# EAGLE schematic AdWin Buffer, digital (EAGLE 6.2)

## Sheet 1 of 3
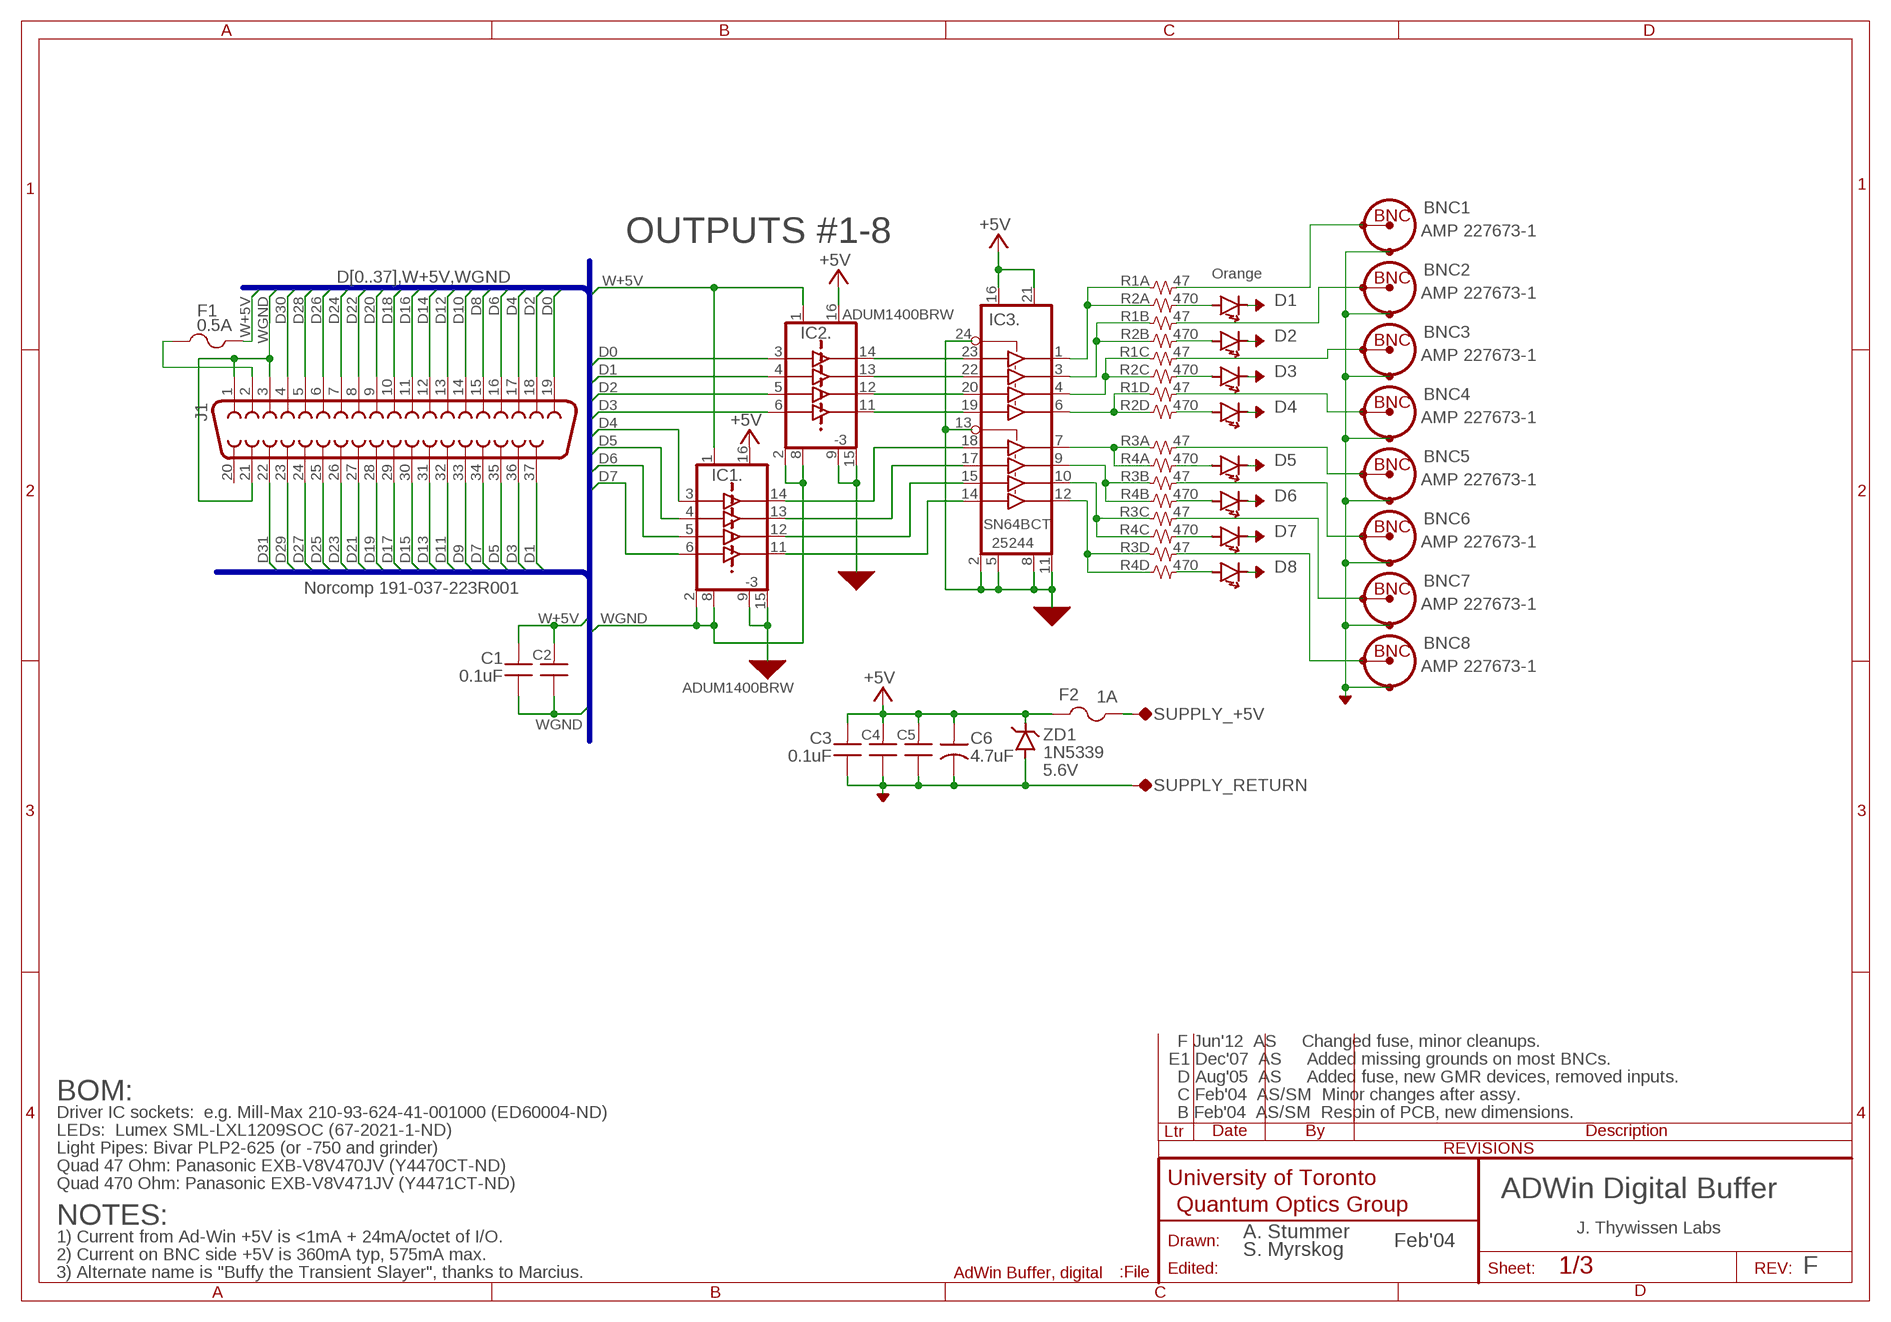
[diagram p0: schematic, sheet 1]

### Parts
BNC1  AMP 227673-1  CONN-BNC-TYPE1VERT  [CONN-BNC-AMP-TYPE1VERT]
BNC2  AMP 227673-1  CONN-BNC-TYPE1VERT  [CONN-BNC-AMP-TYPE1VERT]
BNC3  AMP 227673-1  CONN-BNC-TYPE1VERT  [CONN-BNC-AMP-TYPE1VERT]
BNC4  AMP 227673-1  CONN-BNC-TYPE1VERT  [CONN-BNC-AMP-TYPE1VERT]
BNC5  AMP 227673-1  CONN-BNC-TYPE1VERT  [CONN-BNC-AMP-TYPE1VERT]
BNC6  AMP 227673-1  CONN-BNC-TYPE1VERT  [CONN-BNC-AMP-TYPE1VERT]
BNC7  AMP 227673-1  CONN-BNC-TYPE1VERT  [CONN-BNC-AMP-TYPE1VERT]
BNC8  AMP 227673-1  CONN-BNC-TYPE1VERT  [CONN-BNC-AMP-TYPE1VERT]
C1  0.1uF  CAP-V-0805  [0805]
C2  0.1uF  CAP-V-0805  [0805]
C3  0.1uF  CAP-V-0805  [0805]
C4  0.1uF  CAP-V-0805  [0805]
C5  0.1uF  CAP-V-0805  [0805]
C6  4.7uF  CAP-POL-EIA-B  [EIA-B]
D1  LED-1209  [1209]
D2  LED-1209  [1209]
D3  LED-1209  [1209]
D4  LED-1209  [1209]
D5  LED-1209  [1209]
D6  LED-1209  [1209]
D7  LED-1209  [1209]
D8  LED-1209  [1209]
F1  0.5A  FUSE-5X20-4  [FUSE]
F2  1A  FUSE-5X20-4  [FUSE]
IC1  ADUM1400BRW  ISOLATOR,QUADTTLSOIC-16W  [SOIC-16W]
IC2  ADUM1400BRW  ISOLATOR,QUADTTLSOIC-16W  [SOIC-16W]
IC3  SN64BCT25244NT  LOGIC,BUFFER:64BCT2544(OCTAL)NT  [DIL24]
J1  Norcomp 191-037-223R001  CONN:DB37V  [CONN:DB37-VERT]
R1  47  R-4PAK-0603  [PANASONIC_EXB-V8V(QUAD-R-PACK)]
R2  470  R-4PAK-0603  [PANASONIC_EXB-V8V(QUAD-R-PACK)]
R3  47  R-4PAK-0603  [PANASONIC_EXB-V8V(QUAD-R-PACK)]
R4  470  R-4PAK-0603  [PANASONIC_EXB-V8V(QUAD-R-PACK)]
SUPPLY_+5V  TP-HOLE-0.042  [TP-HOLE]
SUPPLY_RETURN  TP-HOLE-0.042  [TP-HOLE]
ZD1  1N5339  ZENER-EIA-B  [EIA-B]

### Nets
+5V [PowerA]: C3.2 C4.2 C5.2 C6.2(POS) F2.1A IC1.16(.:VDDOUT) IC2.16(.:VDDOUT) IC3.16(.:VDD1) IC3.21(.:VDD2) ZD1.2(C) ; also sheet 2,3
AGND [PowerA]: BNC1.SHIELD BNC2.SHIELD BNC3.SHIELD BNC4.SHIELD BNC5.SHIELD BNC6.SHIELD BNC7.SHIELD BNC8.SHIELD C3.1 C4.1 C5.1 C6.1(NEG) D1.K(C) D2.K(C) D3.K(C) D4.K(C) D5.K(C) D6.K(C) D7.K(C) D8.K(C) IC1.9(.:COM1OUT) IC1.15(.:COM2OUT) IC2.9(.:COM1OUT) IC2.15(.:COM2OUT) IC3.2(.:COM1) IC3.5(.:COM2) IC3.8(.:COM3) IC3.11(.:COM4) IC3.13(.:EN-58) IC3.24(.:EN-14) SUPPLY_RETURN.P$1(TP) ZD1.1(A) ; also sheet 2,3
D0: IC2.3(IN) J1.19
D1: IC2.4(IN) J1.37
D2: IC2.5(IN) J1.18
D3: IC2.6(IN) J1.36
D4: IC1.3(IN) J1.17
D5: IC1.4(IN) J1.35
D6: IC1.5(IN) J1.16
D7: IC1.6(IN) J1.34
D8: J1.15 ; also sheet 2
D9: J1.33 ; also sheet 2
D10: J1.14 ; also sheet 2
D11: J1.32 ; also sheet 2
D12: J1.13 ; also sheet 2
D13: J1.31 ; also sheet 2
D14: J1.12 ; also sheet 2
D15: J1.30 ; also sheet 2
D16: J1.11 ; also sheet 3
D17: J1.29 ; also sheet 3
D18: J1.10 ; also sheet 3
D19: J1.28 ; also sheet 3
D20: J1.9 ; also sheet 3
D21: J1.27 ; also sheet 3
D22: J1.8 ; also sheet 3
D23: J1.26 ; also sheet 3
D24: J1.7 ; also sheet 3
D25: J1.25 ; also sheet 3
D26: J1.6 ; also sheet 3
D27: J1.24 ; also sheet 3
D28: J1.5 ; also sheet 3
D29: J1.23 ; also sheet 3
D30: J1.4 ; also sheet 3
D31: J1.22 ; also sheet 3
N$1: IC2.14(Q) IC3.23(1:IN)
N$2: IC2.13(Q) IC3.22(2:IN)
N$3: IC2.12(Q) IC3.20(3:IN)
N$4: IC2.11(Q) IC3.19(4:IN)
N$7: IC1.11(Q) IC3.14(8:IN)
N$10: IC3.6(4:Q) R1.4A R2.4A
N$11: IC3.4(3:Q) R1.3A R2.3A
N$12: IC3.3(2:Q) R1.2A R2.2A
N$13: IC3.1(1:Q) R1.1A R2.1A
N$14: IC3.7(5:Q) R3.1A R4.1A
N$15: IC3.9(6:Q) R3.2A R4.2A
N$16: IC1.12(Q) IC3.15(7:IN)
N$17: IC1.13(Q) IC3.17(6:IN)
N$18: IC1.14(Q) IC3.18(5:IN)
N$19: IC3.10(7:Q) R3.3A R4.3A
N$20: IC3.12(8:Q) R3.4A R4.4A
N$24: D1.A R2.1B
N$27: D4.A R2.4B
N$28: D3.A R2.3B
N$29: D2.A R2.2B
N$37: D8.A R4.4B
N$39: D7.A R4.3B
N$40: D6.A R4.2B
N$41: D5.A R4.1B
N$49 [Power clearance]: F2.2A SUPPLY_+5V.P$1(TP)
N$58 [PowerA]: F1.1A J1.2
N$123: BNC1.CONDUCTOR R1.1B
N$132: BNC2.CONDUCTOR R1.2B
N$133: BNC3.CONDUCTOR R1.3B
N$134: BNC4.CONDUCTOR R1.4B
N$135: BNC5.CONDUCTOR R3.1B
N$136: BNC6.CONDUCTOR R3.2B
N$137: BNC7.CONDUCTOR R3.3B
N$138: BNC8.CONDUCTOR R3.4B
W+5V [PowerA]: C1.2 C2.2 F1.2A IC1.1(.:VDDIN) IC2.1(.:VDDIN) ; also sheet 2,3
WGND [PowerA]: C1.1 C2.1 IC1.2(.:COM1IN) IC1.8(.:COM2IN) IC2.2(.:COM1IN) IC2.8(.:COM2IN) J1.1 J1.3 J1.21 ; also sheet 2,3
Unconnected: J1.20

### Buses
D[0..37],W+5V,WGND

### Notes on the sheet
- OUTPUTS #1-8
- Orange
- -3
- -3
- 5.6V
- F Jun'12  AS     Changed fuse, minor cleanups.
- E1 Dec'07  AS     Added missing grounds on most BNCs.
- D Aug'05  AS     Added fuse, new GMR devices, removed inputs.
- BOM: | C Feb'04  AS/SM  Minor changes after assy.
- Driver IC sockets:  e.g. Mill-Max 210-93-624-41-001000 (ED60004-ND) | B Feb'04  AS/SM  Respin of PCB, new dimensions.
- LEDs:  Lumex SML-LXL1209SOC (67-2021-1-ND)
- Light Pipes: Bivar PLP2-625 (or -750 and grinder)
- Quad 47 Ohm: Panasonic EXB-V8V470JV (Y4470CT-ND)
- Quad 470 Ohm: Panasonic EXB-V8V471JV (Y4471CT-ND)
- ADWin Digital Buffer
- NOTES:
- A. Stummer | J. Thywissen Labs
- 1) Current from Ad-Win +5V is <1mA + 24mA/octet of I/O. | Feb'04
- 2) Current on BNC side +5V is 360mA typ, 575mA max. | S. Myrskog
- 3) Alternate name is "Buffy the Transient Slayer", thanks to Marcius. | F

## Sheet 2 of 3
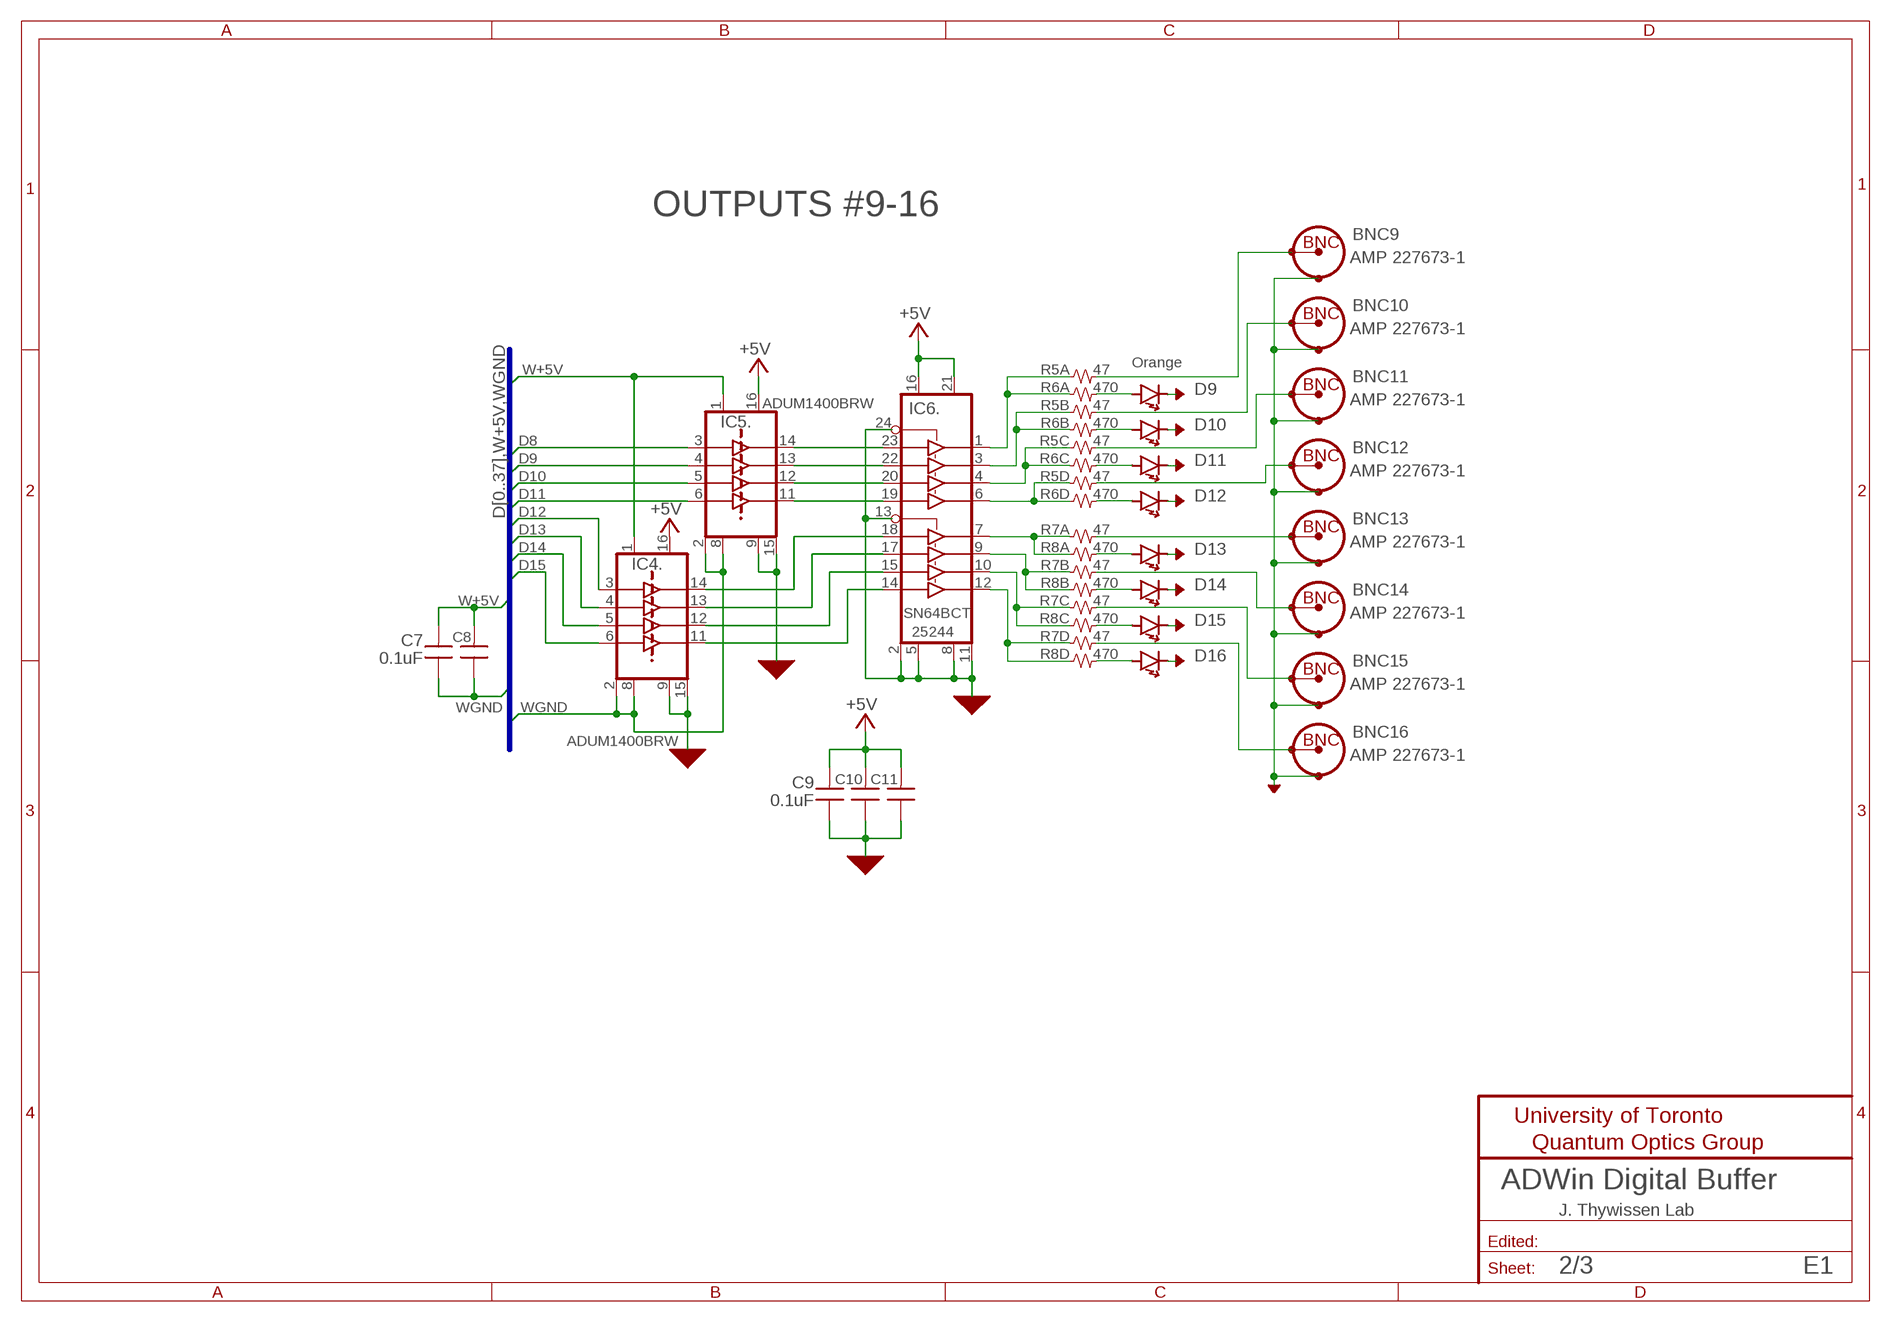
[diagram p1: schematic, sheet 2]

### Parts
BNC9  AMP 227673-1  CONN-BNC-TYPE1VERT  [CONN-BNC-AMP-TYPE1VERT]
BNC10  AMP 227673-1  CONN-BNC-TYPE1VERT  [CONN-BNC-AMP-TYPE1VERT]
BNC11  AMP 227673-1  CONN-BNC-TYPE1VERT  [CONN-BNC-AMP-TYPE1VERT]
BNC12  AMP 227673-1  CONN-BNC-TYPE1VERT  [CONN-BNC-AMP-TYPE1VERT]
BNC13  AMP 227673-1  CONN-BNC-TYPE1VERT  [CONN-BNC-AMP-TYPE1VERT]
BNC14  AMP 227673-1  CONN-BNC-TYPE1VERT  [CONN-BNC-AMP-TYPE1VERT]
BNC15  AMP 227673-1  CONN-BNC-TYPE1VERT  [CONN-BNC-AMP-TYPE1VERT]
BNC16  AMP 227673-1  CONN-BNC-TYPE1VERT  [CONN-BNC-AMP-TYPE1VERT]
C7  0.1uF  CAP-V-0805  [0805]
C8  0.1uF  CAP-V-0805  [0805]
C9  0.1uF  CAP-V-0805  [0805]
C10  0.1uF  CAP-V-0805  [0805]
C11  0.1uF  CAP-V-0805  [0805]
D9  LED-1209  [1209]
D10  LED-1209  [1209]
D11  LED-1209  [1209]
D12  LED-1209  [1209]
D13  LED-1209  [1209]
D14  LED-1209  [1209]
D15  LED-1209  [1209]
D16  LED-1209  [1209]
IC4  ADUM1400BRW  ISOLATOR,QUADTTLSOIC-16W  [SOIC-16W]
IC5  ADUM1400BRW  ISOLATOR,QUADTTLSOIC-16W  [SOIC-16W]
IC6  SN64BCT25244NT  LOGIC,BUFFER:64BCT2544(OCTAL)NT  [DIL24]
R5  47  R-4PAK-0603  [PANASONIC_EXB-V8V(QUAD-R-PACK)]
R6  470  R-4PAK-0603  [PANASONIC_EXB-V8V(QUAD-R-PACK)]
R7  47  R-4PAK-0603  [PANASONIC_EXB-V8V(QUAD-R-PACK)]
R8  470  R-4PAK-0603  [PANASONIC_EXB-V8V(QUAD-R-PACK)]

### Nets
+5V [PowerA]: C9.2 C10.2 C11.2 IC4.16(.:VDDOUT) IC5.16(.:VDDOUT) IC6.16(.:VDD1) IC6.21(.:VDD2) ; also sheet 1,3
AGND [PowerA]: BNC9.SHIELD BNC10.SHIELD BNC11.SHIELD BNC12.SHIELD BNC13.SHIELD BNC14.SHIELD BNC15.SHIELD BNC16.SHIELD C9.1 C10.1 C11.1 D9.K(C) D10.K(C) D11.K(C) D12.K(C) D13.K(C) D14.K(C) D15.K(C) D16.K(C) IC4.9(.:COM1OUT) IC4.15(.:COM2OUT) IC5.9(.:COM1OUT) IC5.15(.:COM2OUT) IC6.2(.:COM1) IC6.5(.:COM2) IC6.8(.:COM3) IC6.11(.:COM4) IC6.13(.:EN-58) IC6.24(.:EN-14) ; also sheet 1,3
D8: IC5.3(IN) ; also sheet 1
D9: IC5.4(IN) ; also sheet 1
D10: IC5.5(IN) ; also sheet 1
D11: IC5.6(IN) ; also sheet 1
D12: IC4.3(IN) ; also sheet 1
D13: IC4.4(IN) ; also sheet 1
D14: IC4.5(IN) ; also sheet 1
D15: IC4.6(IN) ; also sheet 1
N$5: IC5.14(Q) IC6.23(1:IN)
N$6: IC5.13(Q) IC6.22(2:IN)
N$8: IC5.12(Q) IC6.20(3:IN)
N$9: IC5.11(Q) IC6.19(4:IN)
N$21: IC4.11(Q) IC6.14(8:IN)
N$22: IC4.12(Q) IC6.15(7:IN)
N$23: IC4.13(Q) IC6.17(6:IN)
N$25: IC4.14(Q) IC6.18(5:IN)
N$26: IC6.6(4:Q) R5.4A R6.4A
N$30: IC6.4(3:Q) R5.3A R6.3A
N$31: IC6.3(2:Q) R5.2A R6.2A
N$32: IC6.1(1:Q) R5.1A R6.1A
N$33: IC6.7(5:Q) R7.1A R8.1A
N$34: IC6.9(6:Q) R7.2A R8.2A
N$35: IC6.10(7:Q) R7.3A R8.3A
N$36: IC6.12(8:Q) R7.4A R8.4A
N$38: D9.A R6.1B
N$42: D10.A R6.2B
N$43: D11.A R6.3B
N$44: D12.A R6.4B
N$45: D13.A R8.1B
N$46: D14.A R8.2B
N$47: D15.A R8.3B
N$48: D16.A R8.4B
N$124: BNC12.CONDUCTOR R5.4B
N$125: BNC11.CONDUCTOR R5.3B
N$126: BNC10.CONDUCTOR R5.2B
N$127: BNC9.CONDUCTOR R5.1B
N$128: BNC13.CONDUCTOR R7.1B
N$129: BNC16.CONDUCTOR R7.4B
N$130: BNC15.CONDUCTOR R7.3B
N$131: BNC14.CONDUCTOR R7.2B
W+5V [PowerA]: C7.2 C8.2 IC4.1(.:VDDIN) IC5.1(.:VDDIN) ; also sheet 1,3
WGND [PowerA]: C7.1 C8.1 IC4.2(.:COM1IN) IC4.8(.:COM2IN) IC5.2(.:COM1IN) IC5.8(.:COM2IN) ; also sheet 1,3

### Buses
D[0..37],W+5V,WGND

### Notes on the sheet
- OUTPUTS #9-16
- Orange
- ADWin Digital Buffer
- J. Thywissen Lab
- E1

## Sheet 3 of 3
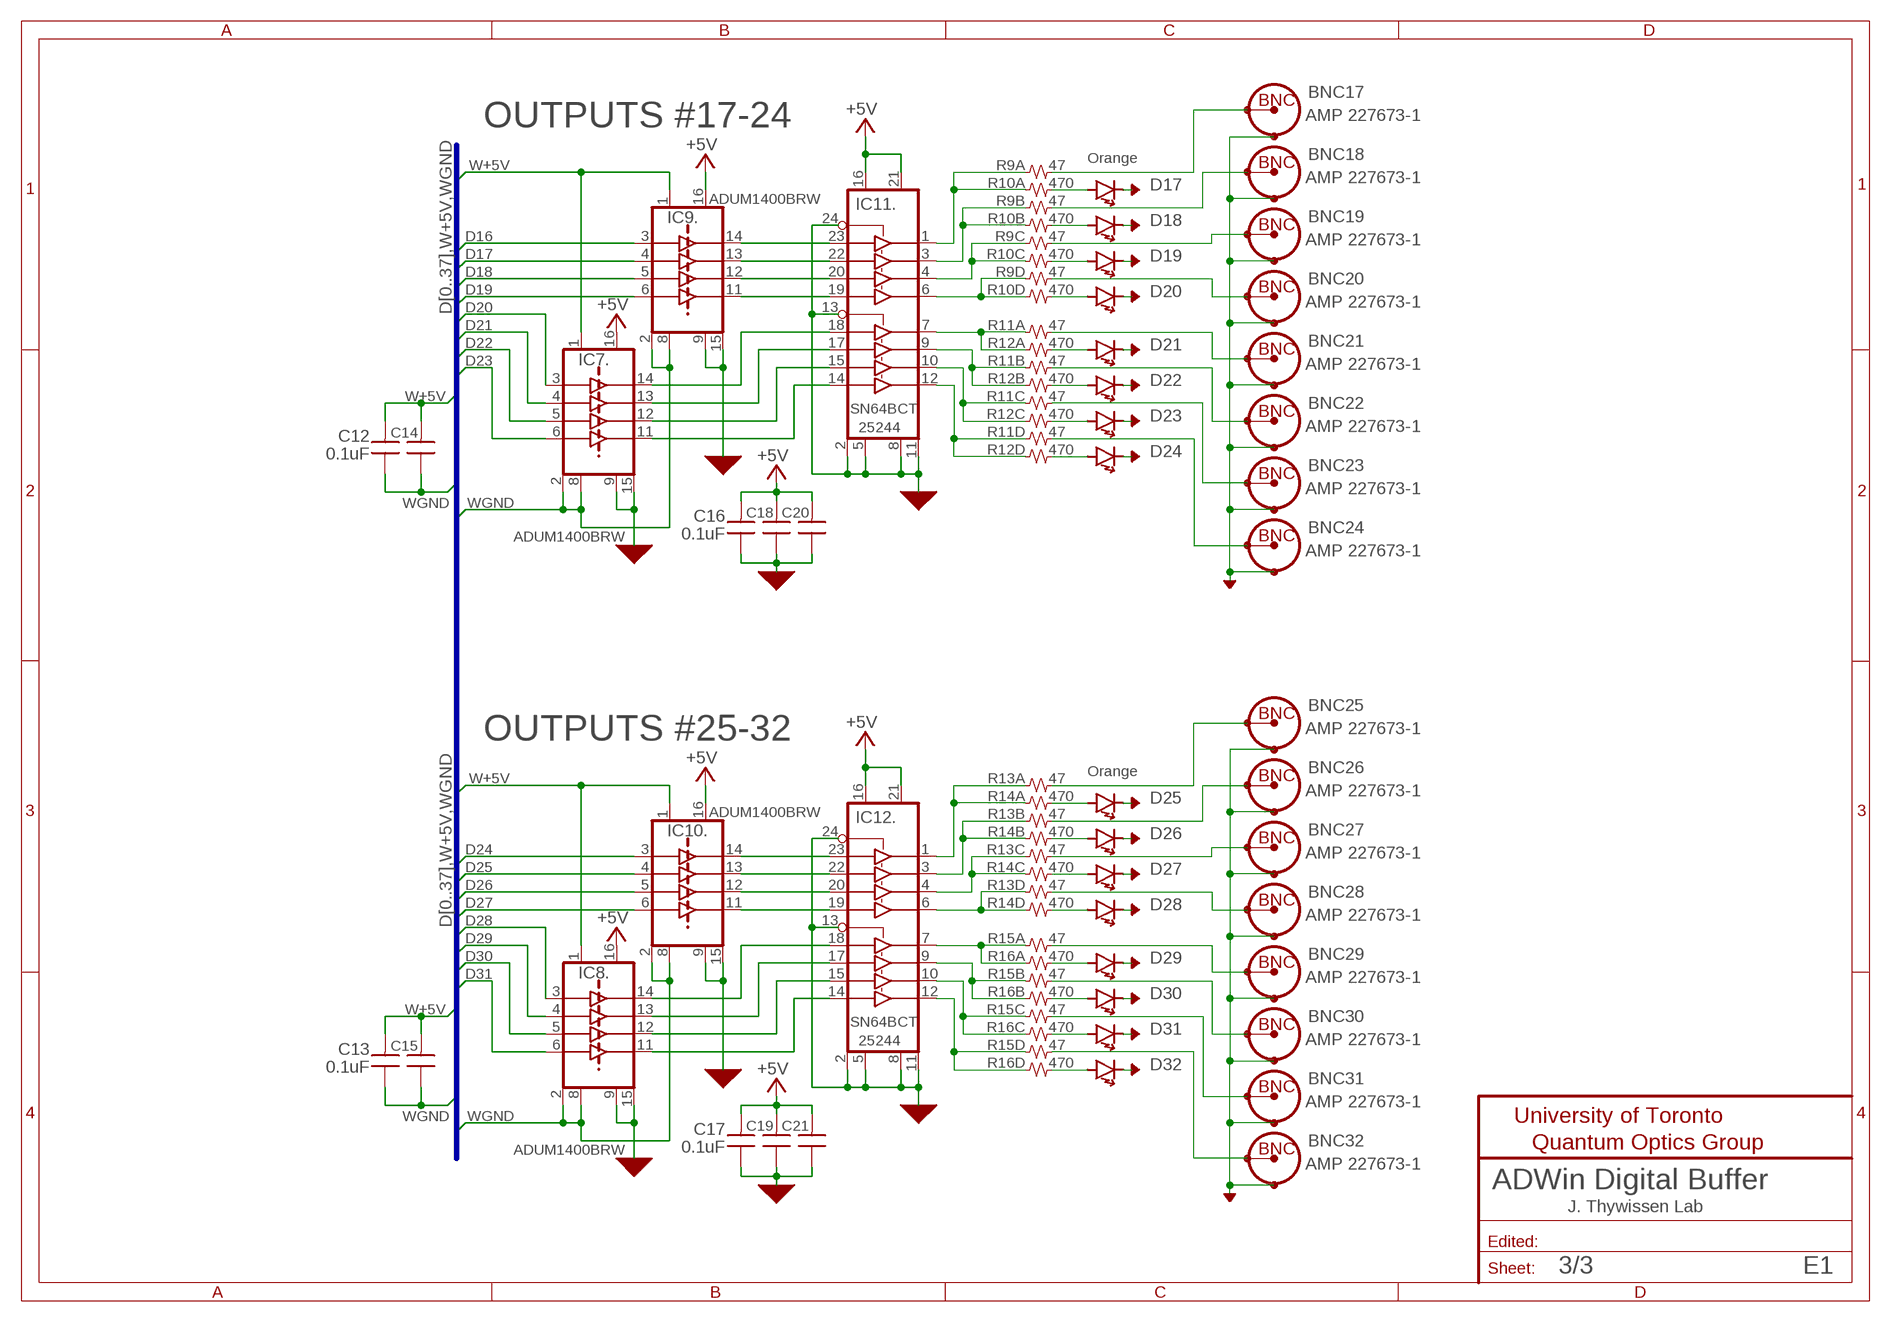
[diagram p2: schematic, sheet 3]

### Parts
BNC17  AMP 227673-1  CONN-BNC-TYPE1VERT  [CONN-BNC-AMP-TYPE1VERT]
BNC18  AMP 227673-1  CONN-BNC-TYPE1VERT  [CONN-BNC-AMP-TYPE1VERT]
BNC19  AMP 227673-1  CONN-BNC-TYPE1VERT  [CONN-BNC-AMP-TYPE1VERT]
BNC20  AMP 227673-1  CONN-BNC-TYPE1VERT  [CONN-BNC-AMP-TYPE1VERT]
BNC21  AMP 227673-1  CONN-BNC-TYPE1VERT  [CONN-BNC-AMP-TYPE1VERT]
BNC22  AMP 227673-1  CONN-BNC-TYPE1VERT  [CONN-BNC-AMP-TYPE1VERT]
BNC23  AMP 227673-1  CONN-BNC-TYPE1VERT  [CONN-BNC-AMP-TYPE1VERT]
BNC24  AMP 227673-1  CONN-BNC-TYPE1VERT  [CONN-BNC-AMP-TYPE1VERT]
BNC25  AMP 227673-1  CONN-BNC-TYPE1VERT  [CONN-BNC-AMP-TYPE1VERT]
BNC26  AMP 227673-1  CONN-BNC-TYPE1VERT  [CONN-BNC-AMP-TYPE1VERT]
BNC27  AMP 227673-1  CONN-BNC-TYPE1VERT  [CONN-BNC-AMP-TYPE1VERT]
BNC28  AMP 227673-1  CONN-BNC-TYPE1VERT  [CONN-BNC-AMP-TYPE1VERT]
BNC29  AMP 227673-1  CONN-BNC-TYPE1VERT  [CONN-BNC-AMP-TYPE1VERT]
BNC30  AMP 227673-1  CONN-BNC-TYPE1VERT  [CONN-BNC-AMP-TYPE1VERT]
BNC31  AMP 227673-1  CONN-BNC-TYPE1VERT  [CONN-BNC-AMP-TYPE1VERT]
BNC32  AMP 227673-1  CONN-BNC-TYPE1VERT  [CONN-BNC-AMP-TYPE1VERT]
C12  0.1uF  CAP-V-0805  [0805]
C13  0.1uF  CAP-V-0805  [0805]
C14  0.1uF  CAP-V-0805  [0805]
C15  0.1uF  CAP-V-0805  [0805]
C16  0.1uF  CAP-V-0805  [0805]
C17  0.1uF  CAP-V-0805  [0805]
C18  0.1uF  CAP-V-0805  [0805]
C19  0.1uF  CAP-V-0805  [0805]
C20  0.1uF  CAP-V-0805  [0805]
C21  0.1uF  CAP-V-0805  [0805]
D17  LED-1209  [1209]
D18  LED-1209  [1209]
D19  LED-1209  [1209]
D20  LED-1209  [1209]
D21  LED-1209  [1209]
D22  LED-1209  [1209]
D23  LED-1209  [1209]
D24  LED-1209  [1209]
D25  LED-1209  [1209]
D26  LED-1209  [1209]
D27  LED-1209  [1209]
D28  LED-1209  [1209]
D29  LED-1209  [1209]
D30  LED-1209  [1209]
D31  LED-1209  [1209]
D32  LED-1209  [1209]
IC7  ADUM1400BRW  ISOLATOR,QUADTTLSOIC-16W  [SOIC-16W]
IC8  ADUM1400BRW  ISOLATOR,QUADTTLSOIC-16W  [SOIC-16W]
IC9  ADUM1400BRW  ISOLATOR,QUADTTLSOIC-16W  [SOIC-16W]
IC10  ADUM1400BRW  ISOLATOR,QUADTTLSOIC-16W  [SOIC-16W]
IC11  SN64BCT25244NT  LOGIC,BUFFER:64BCT2544(OCTAL)NT  [DIL24]
IC12  SN64BCT25244NT  LOGIC,BUFFER:64BCT2544(OCTAL)NT  [DIL24]
R9  47  R-4PAK-0603  [PANASONIC_EXB-V8V(QUAD-R-PACK)]
R10  470  R-4PAK-0603  [PANASONIC_EXB-V8V(QUAD-R-PACK)]
R11  47  R-4PAK-0603  [PANASONIC_EXB-V8V(QUAD-R-PACK)]
R12  470  R-4PAK-0603  [PANASONIC_EXB-V8V(QUAD-R-PACK)]
R13  47  R-4PAK-0603  [PANASONIC_EXB-V8V(QUAD-R-PACK)]
R14  470  R-4PAK-0603  [PANASONIC_EXB-V8V(QUAD-R-PACK)]
R15  47  R-4PAK-0603  [PANASONIC_EXB-V8V(QUAD-R-PACK)]
R16  470  R-4PAK-0603  [PANASONIC_EXB-V8V(QUAD-R-PACK)]

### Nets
+5V [PowerA]: C16.2 C17.2 C18.2 C19.2 C20.2 C21.2 IC7.16(.:VDDOUT) IC8.16(.:VDDOUT) IC9.16(.:VDDOUT) IC10.16(.:VDDOUT) IC11.16(.:VDD1) IC11.21(.:VDD2) IC12.16(.:VDD1) IC12.21(.:VDD2) ; also sheet 1,2
AGND [PowerA]: BNC17.SHIELD BNC18.SHIELD BNC19.SHIELD BNC20.SHIELD BNC21.SHIELD BNC22.SHIELD BNC23.SHIELD BNC24.SHIELD BNC25.SHIELD BNC26.SHIELD BNC27.SHIELD BNC28.SHIELD BNC29.SHIELD BNC30.SHIELD BNC31.SHIELD BNC32.SHIELD C16.1 C17.1 C18.1 C19.1 C20.1 C21.1 D17.K(C) D18.K(C) D19.K(C) D20.K(C) D21.K(C) D22.K(C) D23.K(C) D24.K(C) D25.K(C) D26.K(C) D27.K(C) D28.K(C) D29.K(C) D30.K(C) D31.K(C) D32.K(C) IC7.9(.:COM1OUT) IC7.15(.:COM2OUT) IC8.9(.:COM1OUT) IC8.15(.:COM2OUT) IC9.9(.:COM1OUT) IC9.15(.:COM2OUT) IC10.9(.:COM1OUT) IC10.15(.:COM2OUT) IC11.2(.:COM1) IC11.5(.:COM2) IC11.8(.:COM3) IC11.11(.:COM4) IC11.13(.:EN-58) IC11.24(.:EN-14) IC12.2(.:COM1) IC12.5(.:COM2) IC12.8(.:COM3) IC12.11(.:COM4) IC12.13(.:EN-58) IC12.24(.:EN-14) ; also sheet 1,2
D16: IC9.3(IN) ; also sheet 1
D17: IC9.4(IN) ; also sheet 1
D18: IC9.5(IN) ; also sheet 1
D19: IC9.6(IN) ; also sheet 1
D20: IC7.3(IN) ; also sheet 1
D21: IC7.4(IN) ; also sheet 1
D22: IC7.5(IN) ; also sheet 1
D23: IC7.6(IN) ; also sheet 1
D24: IC10.3(IN) ; also sheet 1
D25: IC10.4(IN) ; also sheet 1
D26: IC10.5(IN) ; also sheet 1
D27: IC10.6(IN) ; also sheet 1
D28: IC8.3(IN) ; also sheet 1
D29: IC8.4(IN) ; also sheet 1
D30: IC8.5(IN) ; also sheet 1
D31: IC8.6(IN) ; also sheet 1
N$59: IC9.14(Q) IC11.23(1:IN)
N$60: IC9.13(Q) IC11.22(2:IN)
N$61: IC9.12(Q) IC11.20(3:IN)
N$62: IC9.11(Q) IC11.19(4:IN)
N$63: IC7.11(Q) IC11.14(8:IN)
N$64: IC7.12(Q) IC11.15(7:IN)
N$65: IC7.13(Q) IC11.17(6:IN)
N$66: IC7.14(Q) IC11.18(5:IN)
N$67: IC11.6(4:Q) R9.4A R10.4A
N$68: IC11.4(3:Q) R9.3A R10.3A
N$69: IC11.3(2:Q) R9.2A R10.2A
N$70: IC11.1(1:Q) R9.1A R10.1A
N$71: IC11.7(5:Q) R11.1A R12.1A
N$72: IC11.9(6:Q) R11.2A R12.2A
N$73: IC11.10(7:Q) R11.3A R12.3A
N$74: IC11.12(8:Q) R11.4A R12.4A
N$75: D17.A R10.1B
N$76: D18.A R10.2B
N$77: D19.A R10.3B
N$78: D20.A R10.4B
N$79: D21.A R12.1B
N$80: D22.A R12.2B
N$81: D23.A R12.3B
N$82: D24.A R12.4B
N$83: IC10.14(Q) IC12.23(1:IN)
N$84: IC10.13(Q) IC12.22(2:IN)
N$85: IC10.12(Q) IC12.20(3:IN)
N$86: IC10.11(Q) IC12.19(4:IN)
N$87: IC8.11(Q) IC12.14(8:IN)
N$88: IC8.12(Q) IC12.15(7:IN)
N$89: IC8.13(Q) IC12.17(6:IN)
N$90: IC8.14(Q) IC12.18(5:IN)
N$91: IC12.6(4:Q) R13.4A R14.4A
N$92: IC12.4(3:Q) R13.3A R14.3A
N$93: IC12.3(2:Q) R13.2A R14.2A
N$94: IC12.1(1:Q) R13.1A R14.1A
N$95: IC12.7(5:Q) R15.1A R16.1A
N$96: IC12.9(6:Q) R15.2A R16.2A
N$97: IC12.10(7:Q) R15.3A R16.3A
N$98: IC12.12(8:Q) R15.4A R16.4A
N$99: D25.A R14.1B
N$100: D26.A R14.2B
N$101: D27.A R14.3B
N$102: D28.A R14.4B
N$103: D29.A R16.1B
N$104: D30.A R16.2B
N$105: D31.A R16.3B
N$106: D32.A R16.4B
N$107: BNC25.CONDUCTOR R13.1B
N$108: BNC32.CONDUCTOR R15.4B
N$109: BNC31.CONDUCTOR R15.3B
N$110: BNC30.CONDUCTOR R15.2B
N$111: BNC29.CONDUCTOR R15.1B
N$112: BNC26.CONDUCTOR R13.2B
N$113: BNC27.CONDUCTOR R13.3B
N$114: BNC28.CONDUCTOR R13.4B
N$115: BNC17.CONDUCTOR R9.1B
N$116: BNC18.CONDUCTOR R9.2B
N$117: BNC19.CONDUCTOR R9.3B
N$118: BNC20.CONDUCTOR R9.4B
N$119: BNC24.CONDUCTOR R11.4B
N$120: BNC23.CONDUCTOR R11.3B
N$121: BNC22.CONDUCTOR R11.2B
N$122: BNC21.CONDUCTOR R11.1B
W+5V [PowerA]: C12.2 C13.2 C14.2 C15.2 IC7.1(.:VDDIN) IC8.1(.:VDDIN) IC9.1(.:VDDIN) IC10.1(.:VDDIN) ; also sheet 1,2
WGND [PowerA]: C12.1 C13.1 C14.1 C15.1 IC7.2(.:COM1IN) IC7.8(.:COM2IN) IC8.2(.:COM1IN) IC8.8(.:COM2IN) IC9.2(.:COM1IN) IC9.8(.:COM2IN) IC10.2(.:COM1IN) IC10.8(.:COM2IN) ; also sheet 1,2

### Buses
D[0..37],W+5V,WGND

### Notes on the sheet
- OUTPUTS #17-24
- Orange
- OUTPUTS #25-32
- Orange
- ADWin Digital Buffer
- J. Thywissen Lab
- E1

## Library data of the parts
BNC1-BNC32 = QuantumOptics:CONN-BNC: BNC PCB connectorsUses 0.1" grid.
C1-C5 C7-C21 = 0-UofT-Physics:CAP-V-: Cap, SMT, 0402 to 1206
C6 = 0-UofT-Physics:CAP-POL-: Capacitor, Polarized, electrolytic (tantalum)l.
D1-D32 = QuantumOptics:LED: LED
F1 F2 = QuantumOptics:FUSE: Fuse
IC1 IC2 IC4 IC5 IC7-IC10 = QuantumOptics:ISOLATOR,QUADTTL: Quad Isolator Analog Devices ADUM1400xxx (alternate NVE's IL715), http://www.analog.com/UploadedFiles/Data_Sheets/1013172531ADuM1400_1_2_c.pdf
IC3 IC6 IC11 IC12 = QuantumOptics:LOGIC,BUFFER:64BCT2544(OCTAL): Octal TTL Buffer, tri-state in two groups, high current 50 Ohm driver.
J1 = QuantumOptics:CONN:DB37: D-Type DB-37
R1-R16 = QuantumOptics:R-4PAK: Quad Resistor Pack
SUPPLY_+5V SUPPLY_RETURN = 0-UofT-Physics:TP: Testpoint, test point on schematic, small pad on PCB.
ZD1 = 0-UofT-Physics:ZENER: Zener

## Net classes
0 default: drill 0.508 mm
1 PowerA: width 0.406 mm, drill 0.711 mm
2 Power clearance: width 0.406 mm, drill 0.711 mm, clearance 0.508 mm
